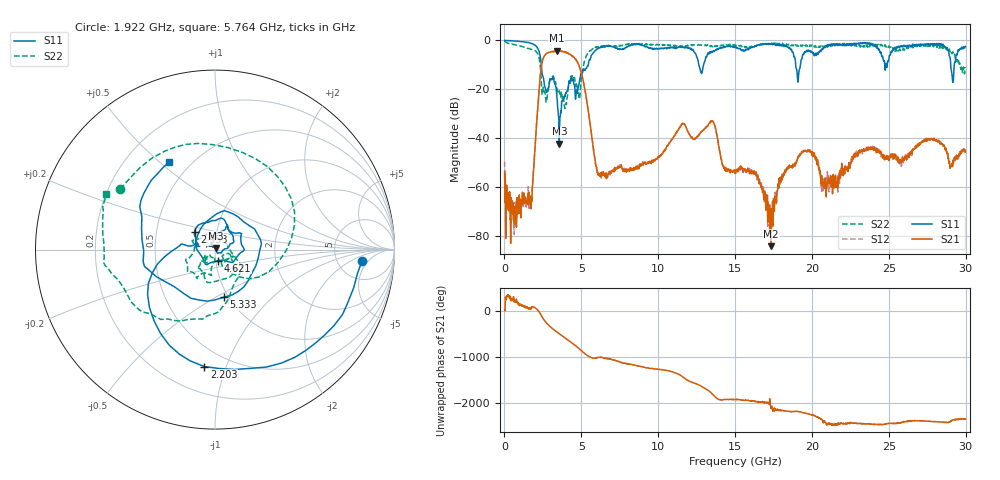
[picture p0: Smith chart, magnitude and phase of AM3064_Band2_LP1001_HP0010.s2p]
# Hz S DB R 50.0
!freq dBS11 angS11 dBS21 angS21 dBS12 angS12 dBS22 angS22
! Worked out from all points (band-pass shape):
!   1600 points, 10 MHz to 29.98 GHz, reference 50 ohm
!   highest |S21| = -4.24 dB at 3.403 GHz (marker M1); lowest = -84.0 dB at 17.35 GHz (marker M2)
!   |S21| within 3 dB of the highest: 2.527 GHz to 4.568 GHz (2.041 GHz wide, 57.5 % of centre)
!   lowest |S11| = -42.1 dB at 3.571 GHz (marker M3), VSWR 1.02, Z = 50.5 + j0.626 ohm
!   |S11| at or under -10 dB: 2.397 GHz to 5.452 GHz (3.055 GHz wide, 77.9 % of centre); 12.64 GHz to 12.95 GHz (308.7 MHz wide, 2.41 % of centre); 18.94 GHz to 19.25 GHz (305.1 MHz wide, 1.6 % of centre)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
!   |S22| runs from -27.8 to -0.3 dB; largest |S21 - S12| = 0.017
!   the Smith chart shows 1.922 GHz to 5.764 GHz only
!   S11 on the Smith chart (normalised r, x): 1.922 GHz: 8.74, -3.47; 2.203 GHz: 0.37, -0.84; 2.953 GHz: 0.78, +0.16; 4.621 GHz: 1.03, -0.13; 5.333 GHz: 0.95, -0.54; 5.764 GHz: 0.38, +0.54
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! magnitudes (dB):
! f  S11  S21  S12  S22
! 10 MHz  0.0  -53.7  -49.3  -0.3
! 684.8 MHz  -0.2  -68.2  -67.0  -1.8
! 1.641 GHz  -1.0  -63.7  -65.2  -3.5
! 1.922 GHz  -1.7  -50.3  -49.7  -4.1
! 2.203 GHz  -3.7  -24.4  -24.3  -5.8
! 2.578 GHz  -17.3  -6.5  -6.5  -21.1
! 2.953 GHz  -16.5  -4.8  -4.8  -15.7
! 3.403 GHz  -22.0  -4.2  -4.3  -19.6
! 3.571 GHz  -42.1  -4.3  -4.3  -20.6
! 4.621 GHz  -24.0  -7.5  -7.6  -18.7
! 5.015 GHz  -13.0  -13.6  -13.6  -14.9
! 5.333 GHz  -11.4  -23.8  -23.9  -6.2
! 5.764 GHz  -5.2  -43.3  -43.0  -3.3
! 6.233 GHz  -2.9  -54.2  -54.9  -2.3
! 10 GHz  -3.4  -47.8  -47.4  -1.8
! 13.49 GHz  -4.5  -32.9  -32.9  -2.3
! 15 GHz  -2.7  -53.9  -53.5  -1.8
! 17.35 GHz  -1.3  -84.0  -72.3  -1.3
! 19.99 GHz  -4.6  -45.7  -45.8  -1.9
! 20.83 GHz  -3.0  -56.3  -58.3  -2.4
! 25 GHz  -8.1  -47.7  -47.1  -2.3
! 29.98 GHz  -2.5  -45.4  -44.4  -10.9
